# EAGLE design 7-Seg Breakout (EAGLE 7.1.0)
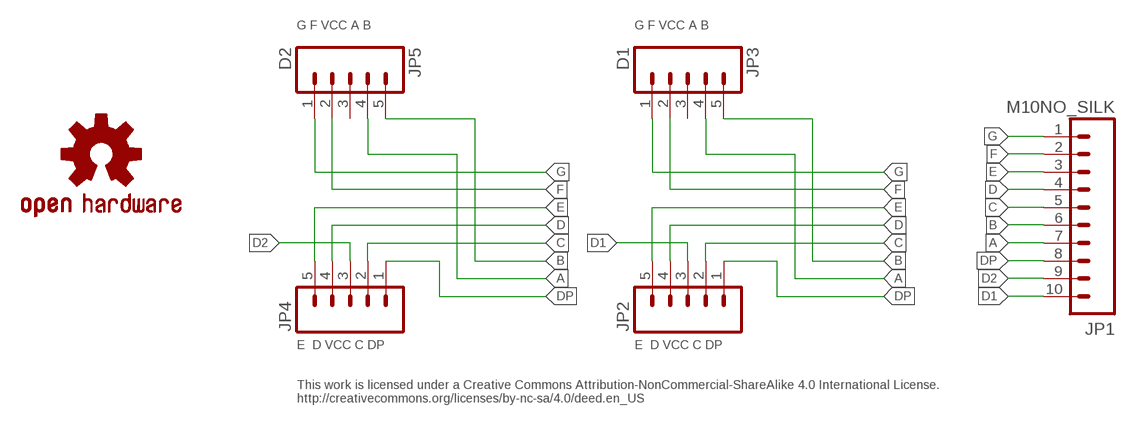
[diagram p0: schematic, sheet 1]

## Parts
JP1  M10NO_SILK  [1X10_NO_SILK]
JP2  M05NO_SILK  [1X05_NO_SILK]
JP3  D1  M05NO_SILK  [1X05_NO_SILK]
JP4  M05NO_SILK  [1X05_NO_SILK]
JP5  D2  M05NO_SILK  [1X05_NO_SILK]
LOGO1  OSHW-LOGOS  [OSHW-LOGO-S]

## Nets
A: JP1.7 JP3.4 JP5.4
B: JP1.6 JP3.5 JP5.5
C: JP1.5 JP2.2 JP4.2
D: JP1.4 JP2.4 JP4.4
D1: JP1.10 JP2.3
D2: JP1.9 JP4.3
DP: JP1.8 JP2.1 JP4.1
E: JP1.3 JP2.5 JP4.5
F: JP1.2 JP3.2 JP5.2
G: JP1.1 JP3.1 JP5.1
Unconnected: JP3.3 JP5.3

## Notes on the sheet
- G F VCC A B | G F VCC A B
- E  D VCC C DP | E  D VCC C DP
- This work is licensed under a Creative Commons Attribution-NonCommercial-ShareAlike 4.0 International License.
  http://creativecommons.org/licenses/by-nc-sa/4.0/deed.en_US

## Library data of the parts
JP1 = SparkFun-Connectors:M10: Header 10 Standard 10-pin 0.1" header. Use with straight break away headers (SKU : PRT-00116), right angle break away headers (PRT-00553), swiss pins (PRT-00743), machine pins (PRT-00117), and female headers (PRT-00115).
JP2-JP5 = SparkFun-Connectors:M05: Header 5 Standard 5-pin 0.1" header. Use with straight break away headers (SKU : PRT-00116), right angle break away headers (PRT-00553), swiss pins (PRT-00743), machine pins (PRT-00117), and female headers (PRT-00115). Molex polarized connector foot print use with SKU : PRT-08230 with associated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
LOGO1 = SparkFun-Aesthetics:OSHW-LOGO: Open Source Hardware Logo This logo indicates the piece of hardware it is found on incorporates a OSHW license and/or adheres to the definition of open source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

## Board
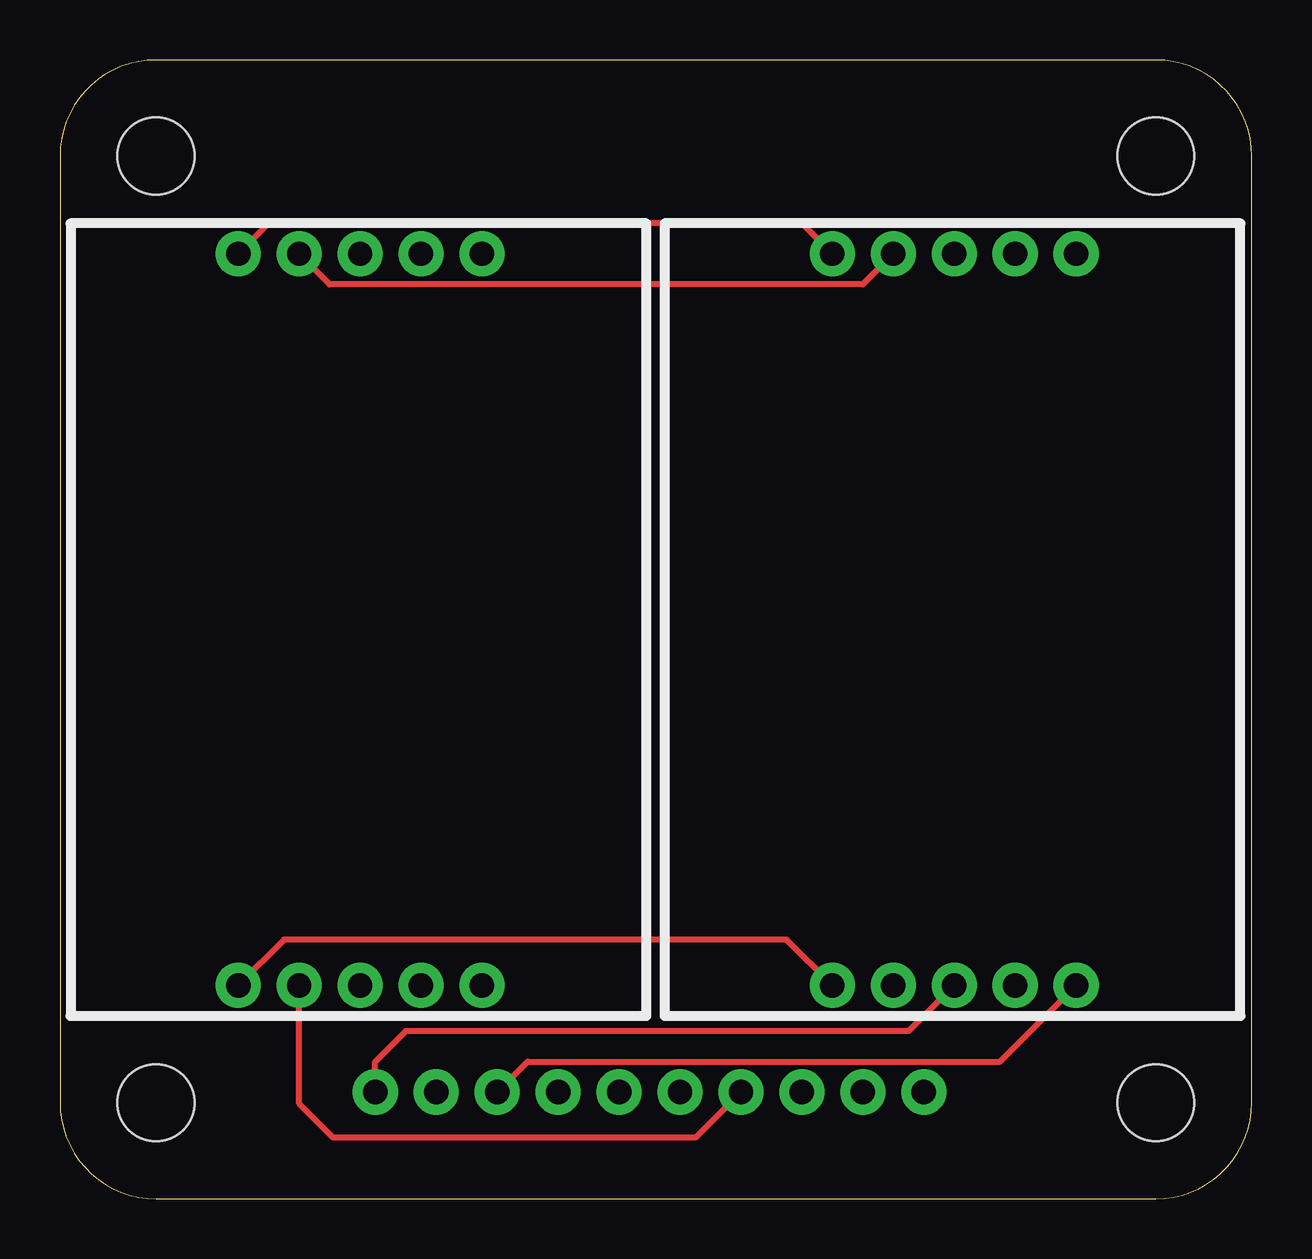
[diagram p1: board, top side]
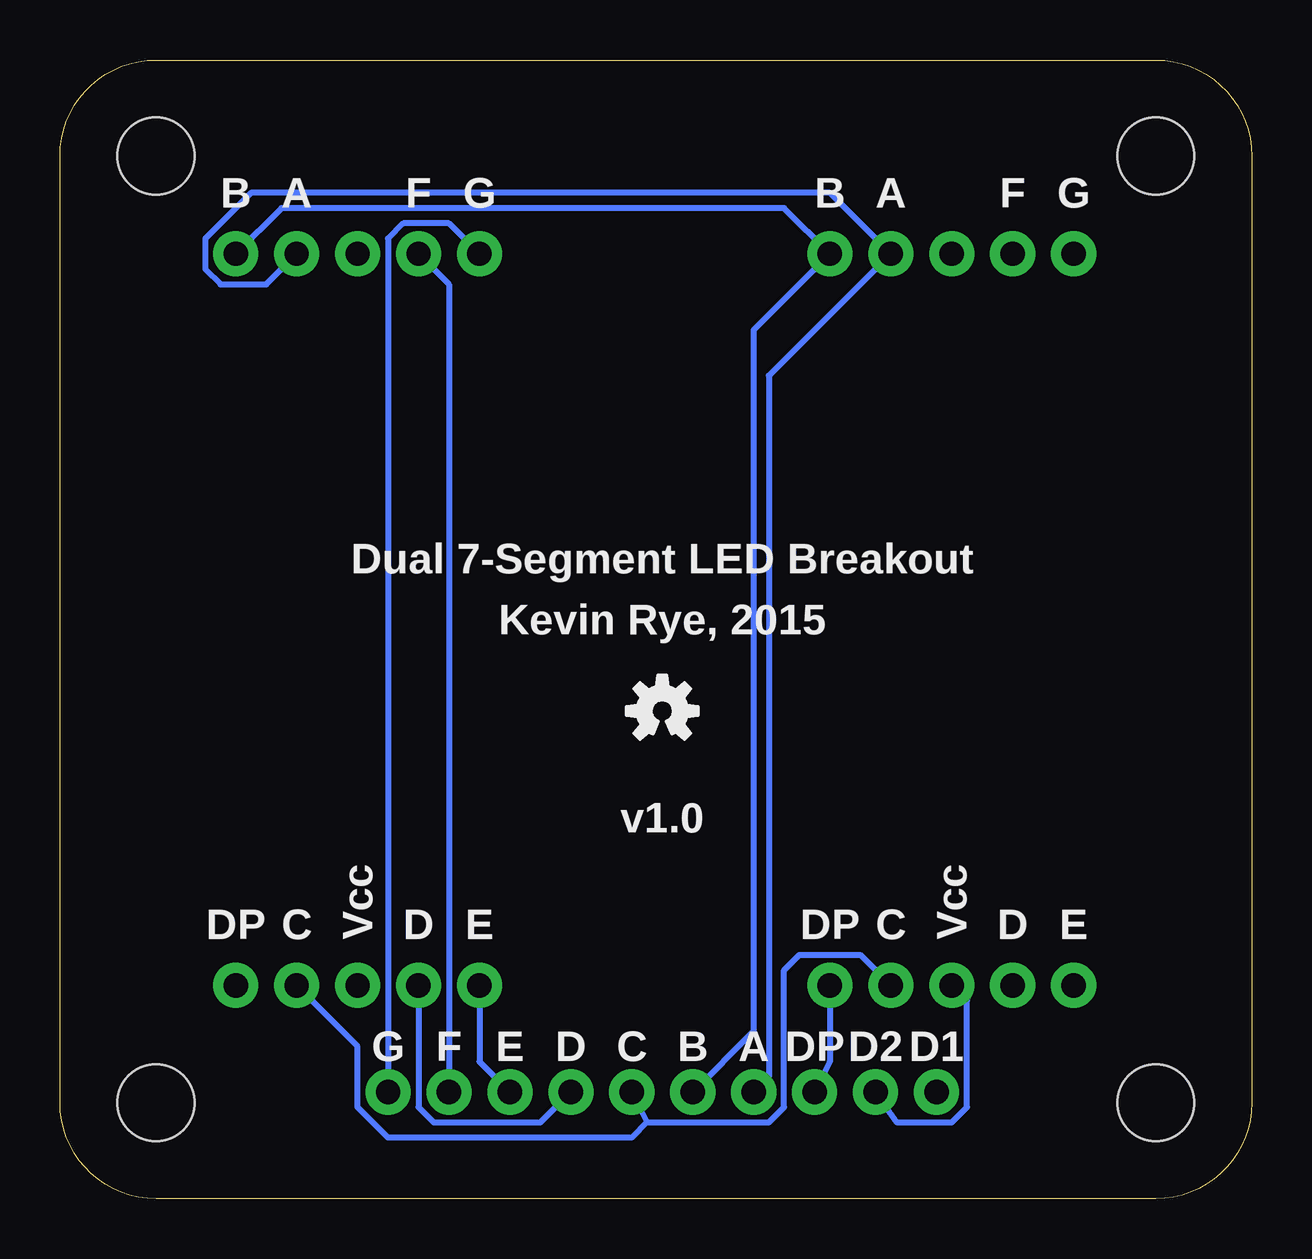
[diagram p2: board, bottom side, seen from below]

Size 49.68 x 47.45 mm. Coordinates in mm from the lower left corner, seen from the top.
Copper layers (1*16): Top 0.035mm / dielectric 1.5mm / Bottom 0.035mm
Design rules "default": minimum track width 10mil, minimum drill 24mil, track to track 8mil, track to pad 8mil, pad to pad 8mil, via to via 8mil, smd to smd 8mil, copper to edge 40mil, drill to drill 8mil, minimum pad ring 10mil, minimum via ring 8mil, stop-mask expansion 4mil, vias tented up to drill 0mil, thermal gap 10mil

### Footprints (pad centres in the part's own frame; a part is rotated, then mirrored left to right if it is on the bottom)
1X10_NO_SILK = drill 1.016 pad 1.88: 1 0,0; 2 2.54,0; 3 5.08,0; 4 7.62,0; 5 10.16,0; 6 12.7,0; 7 15.24,0; 8 17.78,0; 9 20.32,0; 10 22.86,0
1X05_NO_SILK = drill 1.016 pad 1.88: 1 0,0; 2 2.54,0; 3 5.08,0; 4 7.62,0; 5 10.16,0
7-SEGPCB = hole 3.2: 4,2.095; 45.68,2.095; 45.68,41.54; 4,41.54

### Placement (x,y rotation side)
JP1  36,4.45 180 top
JP2  42.35,8.89 180 top
JP3  32.19,39.37 0 top
JP4  17.59,8.89 180 top
JP5  7.43,39.37 0 top
LOGO1  24.57,20.32 0 bottom
U$1  [7-SEGPCB]  0,1.91 0 top

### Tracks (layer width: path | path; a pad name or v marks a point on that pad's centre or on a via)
A
  Bottom 0.254: JP1.7 20.13,5.08 20.13,34.29 JP5.4 17.59,41.91 41.72,41.91 43.62,40.01 43.62,38.73 42.99,38.1 41.08,38.1 JP3.4
B
  Bottom 0.254: JP1.6 20.76,6.99 20.76,36.2 JP5.5 19.49,41.27 40.45,41.27 JP3.5
C
  Bottom 0.254: JP4.2 16.32,10.16 18.86,10.16 19.49,9.53 19.49,3.81 20.13,3.17 25.21,3.17 | JP1.5 25.21,3.17 | JP2.2 37.27,6.35 37.27,3.81 36,2.54 25.84,2.54 25.21,3.17
D
  Top 0.254: JP4.4 9.97,3.96 11.39,2.54 26.48,2.54 JP1.4
  Bottom 0.254: JP1.4 29.65,3.17 34.1,3.17 34.73,3.81 JP2.4
D1
  Top 0.254: JP2.3 35.37,6.99 14.41,6.99 13.14,5.71 JP1.10
D2
  Bottom 0.254: JP4.3 11.87,8.25 11.87,3.81 12.51,3.17 14.79,3.17 JP1.9
DP
  Top 0.254: JP2.1 39.18,5.71 19.49,5.71 JP1.8
  Bottom 0.254: JP4.1 17.59,5.71 JP1.8
E
  Top 0.254: JP4.5 9.33,10.79 30.29,10.79 JP2.5
  Bottom 0.254: JP1.3 32.19,5.71 JP2.5
F
  Top 0.254: JP5.2 11.24,38.1 33.46,38.1 JP3.2
  Bottom 0.254: JP1.2 33.46,38.1 JP3.2
G
  Top 0.254: JP5.1 8.7,40.64 30.92,40.64 JP3.1
  Bottom 0.254: JP1.1 36,40.01 35.37,40.64 33.46,40.64 JP3.1

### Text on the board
Unrouted: This work is licensed under a Creative Commons Attribution-NonCommercial-ShareAlike 4.0 International License. / http://creativecommons.org/licenses/by-nc-sa/4.0/deed.en_US
bNames: G | F | A | B | G | F | A | B | Dual 7-Segment LED Breakout | Kevin Rye, 2015 | v1.0 | E | D | Vcc | C | DP | E | D | Vcc | C | DP | D1 | D2 | DP | A | B | C | D | E | F | G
